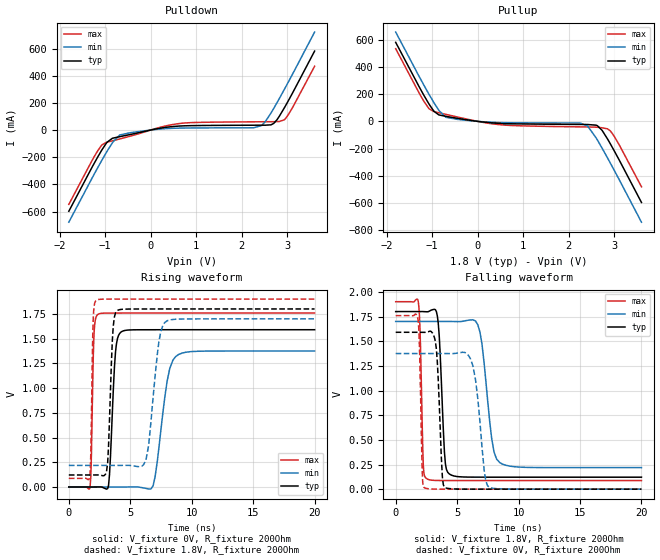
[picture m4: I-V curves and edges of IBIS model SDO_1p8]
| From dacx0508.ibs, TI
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|   Model
[Model]   SDO_1p8
Model_type   Output
Polarity   Non-Inverting
Vmeas = 0.9
Vref = 0
Cref = 1pF
Rref = 100000
|   typ   min   max
C_comp   2.44151pF   1.96628pF   2.93532pF
| Where nom  PVT is Nominal Process, 1.8V, 27C
|   Fast PVT is Strong Process,  1.9V, -40C
|   Slow PVT is Weak Process,   1.7V, 125C
[Voltage Range]   1.8   1.7   1.9
|Junction Temperature
[Temperature Range]   27   125   -40
[Pullup Reference]   1.8   1.7   1.9
[Pulldown Reference]   0   0   0
[Power Clamp Reference]   1.8   1.7   1.9
[GND Clamp Reference]   0   0   0
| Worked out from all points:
|   slope of the pulldown table from 0 to 0.27 V, typ, clamps not added: 16 ohm
|   slope of the pullup table from 0 to 0.27 V, typ, clamps not added: 27.5 ohm
|   falling waveform, V_fixture 1.8V, R_fixture 200Ohm: 20-80 % time 354ps typ, 729ps min, 196ps max; typ from 1.8 V to 0.122 V
|   rising waveform, V_fixture 0V, R_fixture 200Ohm: 20-80 % time 354ps typ, 835ps min, 170ps max; typ from 0 V to 1.59 V
|   rising waveform, V_fixture 1.8V, R_fixture 200Ohm: 20-80 % time 290ps typ, 695ps min, 142ps max; typ from 0.122 V to 1.8 V
|   falling waveform, V_fixture 0V, R_fixture 200Ohm: 20-80 % time 322ps typ, 631ps min, 184ps max; typ from 1.59 V to 0 V
[Pulldown]
|   Voltage   I(typ)   I(min)   I(max)
-1.8V     -598.2mA   -678.6mA   -547.7mA
-1.292V   -275.9mA   -356.1mA   -226.2mA
-1.076V   -148mA     -224.2mA   -111.2mA
-957.6mV  -89.38mA   -155.2mA   -89.16mA
-682.2mV  -49mA      -36.78mA   -65.97mA
651.6mV   29.67mA    14.25mA    48.73mA
2.261V    35.45mA    16.64mA    60.5mA
2.439V    35.66mA    33.11mA    60.91mA
2.704V    48.95mA    160mA      61.53mA
2.941V    166.7mA    302.6mA    77.33mA
3.13V     281.7mA    420.7mA    174.1mA
3.6V      581.1mA    721.1mA    469.6mA
[Pullup]
|   Voltage   I(typ)   I(min)   I(max)
-1.8V     581.7mA    657.2mA    534.8mA
-1.287V   256.2mA    331.9mA    209.8mA
-1.071V   129mA      200.8mA    94.66mA
-855mV    48.15mA    82.85mA    63.7mA
-698.4mV  36.92mA    30.17mA    51.56mA
516.6mV   -15.52mA   -9.275mA   -25.37mA
2.25V     -22.78mA   -12.99mA   -40.55mA
2.417V    -23.3mA    -34.6mA    -41.2mA
2.633V    -32.27mA   -138.4mA   -43.76mA
2.92V     -167.6mA   -309.4mA   -71.58mA
3.119V    -290mA     -434.6mA   -178.1mA
3.6V      -596.9mA   -742.4mA   -481.7mA
[Ramp]
R_load = 200
|   typ   min   max
dV/dt_r   0.95405/3.5442e-10   0.82486/8.34604e-10   1.05536/1.69955e-10
dV/dt_f   1.00705/3.53833e-10   0.888944/7.28623e-10   1.08761/1.96409e-10
[Falling Waveform]
V_fixture = 1.8V
V_fixture_min = 1.7V
V_fixture_max = 1.9V
R_fixture = 200Ohm
C_fixture = 0F
|   Time   V(typ)   V(min)   V(max)
0s        1.8V       1.7V       1.9V
1.833ns   1.8V       1.7V       1.905V
2.246ns   1.8V       1.7V       246mV
2.499ns   1.798V     1.7V       108.7mV
3.389ns   1.756V     1.7V       88.14mV
3.965ns   380.5mV    1.7V       87.58mV
4.321ns   158.9mV    1.7V       87.53mV
6.686ns   121.8mV    1.666V     87.35mV
8.47ns    121.6mV    269.3mV    87.34mV
20ns      121.6mV    218.4mV    87.3mV
[Rising Waveform]
V_fixture = 0V
V_fixture_min = 0V
V_fixture_max = 0V
R_fixture = 200Ohm
C_fixture = 0F
|   Time   V(typ)   V(min)   V(max)
0s        13.64uV    24.04uV    7.902uV
1.735ns   -46.57uV   -63.63nV   5.962mV
2.063ns   -57.96uV   -4.627uV   1.572V
2.378ns   965.6uV    -8.995uV   1.746V
3.234ns   17.07mV    -20.9uV    1.758V
3.8ns     1.364V     -28.76uV   1.759V
4.234ns   1.565V     -34.78uV   1.759V
6.857ns   1.59V      12.3mV     1.759V
8.941ns   1.59V      1.34V      1.759V
20ns      1.59V      1.375V     1.759V
[Rising Waveform]
V_fixture = 1.8V
V_fixture_min = 1.7V
V_fixture_max = 1.9V
R_fixture = 200Ohm
C_fixture = 0F
|   Time   V(typ)   V(min)   V(max)
0s        121.6mV    218.4mV    87.3mV
1.695ns   121.5mV    218.4mV    94.63mV
1.984ns   121.6mV    218.4mV    1.687V
2.246ns   121.9mV    218.4mV    1.888V
3.065ns   152.8mV    218.4mV    1.899V
3.618ns   1.628V     218.4mV    1.9V
3.965ns   1.785V     218.4mV    1.9V
6.277ns   1.8V       272.5mV    1.9V
7.808ns   1.8V       1.663V     1.9V
20ns      1.8V       1.7V       1.9V
[Falling Waveform]
|Gnd
V_fixture = 0V
V_fixture_min = 0V
V_fixture_max = 0V
R_fixture = 200Ohm
C_fixture = 0F
|   Time   V(typ)   V(min)   V(max)
0s        1.59V      1.375V     1.759V
1.792ns   1.59V      1.375V     1.738V
1.914ns   1.59V      1.375V     1.522V
2.158ns   1.59V      1.375V     185mV
2.332ns   1.589V     1.375V     15.22mV
3.234ns   1.495V     1.375V     747.7uV
3.965ns   19.14mV    1.375V     210.3uV
6.277ns   275.8uV    1.253V     56.53uV
7.653ns   99.64uV    15.4mV     51.64uV
20ns      13.67uV    24.43uV    7.768uV
